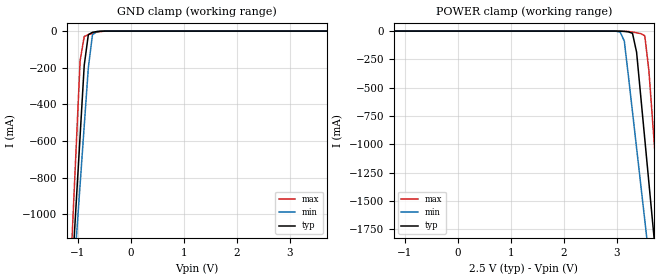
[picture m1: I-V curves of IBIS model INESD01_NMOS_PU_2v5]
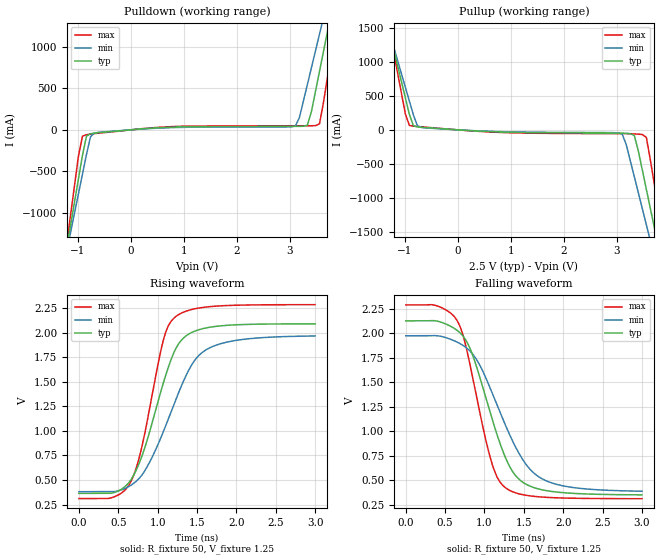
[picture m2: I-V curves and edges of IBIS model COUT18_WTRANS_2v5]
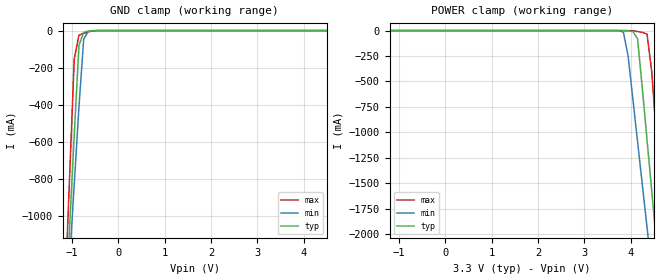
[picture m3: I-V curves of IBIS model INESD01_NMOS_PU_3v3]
|   This file is an IBIS representation of the   |
|   Integrated Device Technology Inc   |
|   ICS840001-34   |
|   FEMTOCLOCKS CRYSTAL-TOLVCMOS/ LVTTL FREQUENCY SYNTHESIZER   |
[IBIS Ver]   4.1
[File name]   840001_34.ibs
[File Rev]   1.0
[Date]   15 Jun 2009 | Last modified
[Source]   Originated at Integrated Devices Technology, Inc.
[Disclaimer]
IDT hereby grants the user of this IBIS model a non-exclusive,
nontransferable license to use this IBIS model under the following terms.
Before using this IBIS model, the user should read this license.
If the user does not accept these terms,  the IBIS model should be
returned to IDT within 30 days.
   The user is granted this license only to use the IBIS model and
is not granted rights to sell, load, rent, lease or license the IBIS
model in whole or in part, or in modified form to anyone other than
user. User may modify the IBIS model to suit its specific
applications but rights to derivative works and such modifications
shall belong to IDT.
   This IBIS model is provided on an "AS IS" basis and IDT makes
absolutely no warranty with respect to the information contained
herein. IDT DISCLAIMS AND CUSTOMER WAIVES ALL WARRANTIES, EXPRESS
OR IMPLIED, INCLUDING WARRANTIES OF MERCHANTABILITY OR FITNESS FOR
A PARTICULAR PURPOSE. The entire risk as to quality and performance
is with the Customer. ACCORDINGLY, IN NO EVENT SHALL THE COMPANY BE
LIABLE FOR ANY DAMAGES, WHETHER IN CONTRACT OR TORT,INCLUDING ANY
LOST PROFITS OR OTHER INCIDENTAL, CONSEQUENTIAL, EXEMPLARY, OR
PUNITIVE DAMAGES ARISING OUT OF THE USE OR APPLICATION OF THE IBIS
model provided in this package. Further, IDT reserves the right to
make changes without notice to any product herein to improve
reliability, function, or design. IDT does not convey any license
under patent rights or any other intellectual property rights,
including those of third parties.
   IDT is not obligated to provide maintenance or support
for the licensed IBIS model.
[Copyright]   Copyright 2005 by IDT Inc.
[Component]   ICS840001K-34
[Manufacturer] Integrated Devices Technology, Inc.
[Package]
|QFN 16
|lead + wire   typ   min   max
R_pkg   72.4655m   58.886m   86.045m
L_pkg   1.47175nH   1.11650nH   1.77850n
C_pkg   0.07747pF   0.07444pF   0.08050pF
[Pin] signal_name  model_name   R_pin   L_pin   C_pin
1   OE   INESD01_NMOS_PU   86.045m   1.77850nH   0.08050pF
2   XTAL_IN   NC   58.886m   1.11650nH   0.07444pF
3   XTAL_OUT   NC   58.886m   1.11650nH   0.07444pF
4   M0   INESD01_NMOS_PU   86.045m   1.77850nH   0.08050pF
5   M1   INESD01_NMOS_PU   86.045m   1.77850nH   0.08050pF
6   NC   NC   58.886m   1.11650nH   0.07444pF
7   N0   INESD01_NMOS_PU   58.886m   1.11650nH   0.07444pF
8   N1   INESD01_NMOS_PU   86.045m   1.77850nH   0.08050pF
9   VDD   POWER   86.045m   1.77850nH   0.08050pF
10   GND   GND   58.886m   1.11650nH   0.07444pF
11   VDD0   POWER   58.886m   1.11650nH   0.07444pF
12   Q   COUT18_WTRANS   86.045m   1.77850nH   0.08050pF
13   REF_OUT   COUT18_WTRANS   86.045m   1.77850nH   0.08050pF
14   NC   NC   58.886m   1.11650nH   0.07444pF
15   NC   NC   58.886m   1.11650nH   0.07444pF
16   VDDA   POWER   86.045m   1.77850nH   0.08050pF
[Model Selector] INESD01_NMOS_PU
INESD01_NMOS_PU_2v5  Buffer selection for 2v5
INESD01_NMOS_PU_3v3  Buffer selection for 3v3
[Model Selector] COUT18_WTRANS
COUT18_WTRANS_2v5  Buffer selection for 2v5
COUT18_WTRANS_3v3  Buffer selection for 3v3
| Models and submodels in the file (4): INESD01_NMOS_PU_2v5 (Input), COUT18_WTRANS_2v5 (Output), INESD01_NMOS_PU_3v3 (Input), COUT18_WTRANS_3v3 (Output)
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[Model] INESD01_NMOS_PU_2v5
Model_type   Input
Polarity   Non-Inverting
Vinl = 0.5V
Vinh = 1.1V
|   typ   min   max
C_comp   2pF   1.5pF   2.5pF
|   typ   min   max
[Voltage range]  2.5V   2.375V   2.625V
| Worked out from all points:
|   GND clamp passes 1 mA (typ) near -0.57 V on its own axis
[GND_clamp]
|Voltage I(typ)   I(min)   I(max)
-2.5V     -8.263A    -7.237A    -9.981A
-1.108V   -1.337A    -1.473A    -1.142A
-1.031V   -953.1mA   -1.154A    -651.2mA
-953.6mV  -569.5mA   -835mA     -160.3mA
-876.3mV  -186.2mA   -516.8mA   -29.47mA
-799mV    -19.59mA   -199.2mA   -19.31mA
-721.6mV  -6.713mA   -20.65mA   -12.35mA
-644.3mV  -2.945mA   -2.694mA   -6.489mA
-489.7mV  -219.7uA   -96.65uA   -544uA
5V        555.4pA    974.3pA    139.3pA
[POWER_clamp]
|Voltage   I(typ)   I(min)   I(max)
-2.5V     555.4pA    852.5pA    162.9pA
3.067V    -971.3uA   -8.981mA   -175.9uA
3.144V    -2.945mA   -87.2mA    -1.018mA
3.299V    -19.59mA   -713mA     -8.571mA
3.376V    -186.2mA   -1.031A    -14.91mA
3.454V    -569.5mA   -1.35A     -22.33mA
3.531V    -953.1mA   -1.669A    -41.51mA
3.608V    -1.337A    -1.989A    -348.5mA
3.686V    -1.721A    -2.309A    -839.4mA
3.763V    -2.106A    -2.628A    -1.33A
3.84V     -2.49A     -2.948A    -1.822A
5V        -8.263A    -7.755A    -9.188A
[Model] COUT18_WTRANS_2v5
Model_type   Output
Polarity   Non-Inverting
|   typ   min   max
C_comp   2pF   1.5pF   2.5pF
Vmeas = 1.25V
Rref = 50
Cref = 0
Vref = 1.25V
|   typ   min   max
[Voltage range]   2.5V   2.375V   2.625V
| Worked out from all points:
|   slope of the pulldown table from 0 to 0.375 V, typ, clamps not added: 19.6 ohm
|   slope of the pullup table from 0 to 0.375 V, typ, clamps not added: 21.5 ohm
|   rising waveform, R_fixture 50, V_fixture 1.25: 20-80 % time 395ps typ, 507ps min, 303ps max; typ from 0.364 V to 2.09 V
|   falling waveform, R_fixture 50, V_fixture 1.25: 20-80 % time 428ps typ, 539ps min, 325ps max; typ from 2.12 V to 0.35 V
[Pulldown]
|Voltage   I (typ)   I (min)   I (max)
-2.5V     -6.273A    -5.512A    -7.555A
-1.212V   -1.443A    -1.481A    -1.401A
-1.136V   -1.158A    -1.244A    -1.039A
-909.1mV  -305.1mA   -532.1mA   -75.35mA
-833.3mV  -76mA      -295.2mA   -58.33mA
-681.8mV  -39.32mA   -38.12mA   -45.27mA
3.106V    41.58mA    46.68mA    48.58mA
3.333V    57.56mA    549mA      48.9mA
3.561V    704.8mA    1.153A     72.58mA
3.712V    1.188A     1.557A     639.5mA
3.864V    1.673A     1.961A     1.257A
5V        5.321A     5.003A     5.911A
[Pullup]
|Voltage   I (typ)   I (min)   I (max)
-2.5V     5.353A     4.699A     6.458A
-1.288V   1.448A     1.44A      1.48A
-984.8mV  472mA      626.4mA    235.1mA
-909.1mV  228.1mA    423mA      64.88mA
-681.8mV  37.67mA    34.77mA    44.41mA
3.106V    -48.75mA   -64.15mA   -56.2mA
3.333V    -82.9mA    -689.3mA   -59.94mA
3.485V    -592.6mA   -1.161A    -68.81mA
3.561V    -875.3mA   -1.397A    -111.4mA
3.712V    -1.441A    -1.869A    -804.5mA
3.864V    -2.008A    -2.342A    -1.527A
5V        -6.261A    -5.891A    -6.948A
[Ramp]
|   typ   min   max
dV/dt_r   1.381/0.608n   1.269/0.793n   1.58/0.474n
dV/dt_f   1.42/0.669n   1.269/0.851n   1.582/0.499n
R_load =   50.0000
[Rising Waveform]
R_fixture = 50
V_fixture = 1.25   |Vcc_typ
V_fixture_min = 1.1875 |Vcc_min
V_fixture_max = 1.3125 |Vcc_max
C_fixture = 0.0p
| Time   typ   min   max
0s        364.1mV    381.2mV    311.1mV
420.4ps   367mV      380.9mV    321.2mV
654.7ps   494.9mV    443.6mV    475.7mV
798.8ps   739.7mV    549.4mV    833.9mV
1.075ns   1.495V     997mV      1.931V
1.225ns   1.829V     1.307V     2.161V
1.45ns    2.009V     1.695V     2.24V
1.673ns   2.058V     1.851V     2.267V
2.132ns   2.085V     1.937V     2.283V
3ns       2.091V     1.968V     2.286V
[Falling Waveform]
R_fixture = 50
V_fixture = 1.25   |Vcc_typ
V_fixture_min = 1.1875 |Vcc_min
V_fixture_max = 1.3125 |Vcc_max
C_fixture = 0.0p
| Time   typ   min   max
0s        2.124V     1.972V     2.286V
393.4ps   2.122V     1.973V     2.278V
660.7ps   2.022V     1.904V     2.115V
738.7ps   1.957V     1.868V     1.945V
831.8ps   1.813V     1.803V     1.617V
1.078ns   1.173V     1.427V     716.2mV
1.258ns   745.4mV    1.075V     428.3mV
1.447ns   503.3mV    760.6mV    359mV
1.754ns   398.3mV    505.1mV    326.6mV
3ns       350.4mV    387.3mV    311.4mV
[Model] INESD01_NMOS_PU_3v3
Model_type   Input
Polarity   Non-Inverting
Vinl = 0.7V
Vinh = 1.3V
|   typ   min   max
C_comp   2pF   1.5pF   2.5pF
|   typ   min   max
[Voltage range]  3.3V   3.15V   3.45V
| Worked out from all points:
|   GND clamp passes 1 mA (typ) near -0.56 V on its own axis
[GND_clamp]
|Voltage   I(typ)   I(min)   I(max)
-3.3V     -12.24A    -10.56A    -15.06A
-1.157V   -1.578A    -1.673A    -1.45A
-1.055V   -1.071A    -1.251A    -801.8mA
-952.6mV  -564.4mA   -830.8mA   -154mA
-850.5mV  -79.92mA   -410.9mA   -24.97mA
-748.5mV  -8.956mA   -45.87mA   -14.66mA
-646.4mV  -3.019mA   -2.828mA   -6.626mA
-544.3mV  -652uA     -309.6uA   -1.636mA
6.6V      4.435nA    6.865nA    1.283nA
[POWER_clamp]
|Voltage   I(typ)   I(min)   I(max)
-3.3V     4.435nA    5.64nA     1.609nA
3.64V     -5.052uA   -135.1uA   -13.25nA
3.844V    -652uA     -14.51mA   -32.02uA
3.946V    -3.019mA   -250.2mA   -451.4uA
4.048V    -8.956mA   -669.7mA   -3.083mA
4.151V    -79.92mA   -1.09A     -9.442mA
4.355V    -1.071A    -1.933A    -33.35mA
4.457V    -1.578A    -2.355A    -402.1mA
4.559V    -2.085A    -2.777A    -1.05A
4.661V    -2.593A    -3.199A    -1.698A
4.763V    -3.101A    -3.622A    -2.347A
6.6V      -12.24A    -11.24A    -14.01A
